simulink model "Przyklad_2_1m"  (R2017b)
settings: Solver=ode45  StartTime=0.0  StopTime=0.05  FixedStep=0.0001  MaxStep=0.0001  RelTol=1e-5  AbsTol=1e-6  EnableMultiTasking=on
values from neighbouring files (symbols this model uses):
  A = [-R2/L 0;0 -1/(R1*(C1+C2))]    [Przyklad_2_1.m]    (also in Przyklad_zs_1.m = [-(1/(R1*C1)+1/(R2*C1)) 1/(R2*C1))
  B = [-A(1,1) 0; 1/(C1+C2) -C2*A(2,2)/(C1+C2)]    [Przyklad_2_1.m]
  C = [1 0;0 -C1*A(2,2);0 C2*A(2,2)]    [Przyklad_2_1.m]
  D = [0 0;-C1*B(2,1) -C1*B(2,2); C2*B(2,1) C2*B(2,2)]    [Przyklad_2_1.m]
  D1 = [0 0;0 -C2*D(2,1);0 C1*D(3,1)]    [Przyklad_2_1.m]

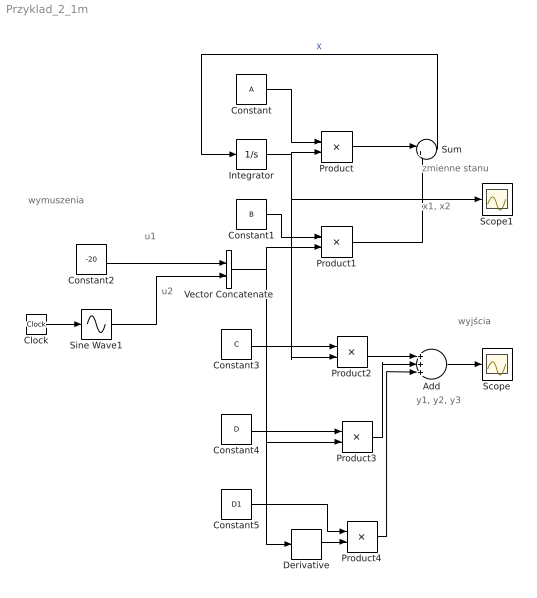
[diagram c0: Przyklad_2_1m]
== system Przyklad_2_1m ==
  note: x1, x2
  note: y1, y2, y3
  note: u2
  note: u1
  note: wymuszenia
  note: wyjścia
  note: zmienne stanu
  Add : Sum  Inputs=+++  SampleTime=0
  Clock : Clock
  Constant : Constant  Value=A  VectorParams1D=off
  Constant1 : Constant  Value=B  VectorParams1D=off
  Constant2 : Constant  Value=-20
  Constant3 : Constant  Value=C  VectorParams1D=off
  Constant4 : Constant  Value=D  VectorParams1D=off
  Constant5 : Constant  Value=D1  VectorParams1D=off
  Derivative : Derivative
  Integrator : Integrator
  Product{,1..4} (5 alike) : Product  Multiplication=Matrix(*)
  Scope : Scope
  Scope1 : Scope
  Sine Wave1 : Sin  TimeSource=Use external signal  Amplitude=50  Frequency=100*pi  SampleTime=0
  Sum : Sum  Inputs=|++
  Vector Concatenate : Concatenate  ConcatenateDimension=2
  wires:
  Integrator/1 -> Product/2, Product2/2, Scope1/1
  Constant/1 -> Product/1
  Constant1/1 -> Product1/1
  Clock/1 -> Sine Wave1/1
  Vector Concatenate/1 -> Product1/2, Derivative/1, Product3/2
  Constant3/1 -> Product2/1
  Derivative/1 -> Product4/2
  Constant5/1 -> Product4/1
  Product/1 -> Sum/1
  Sum/1 -> Integrator/1  "X"
  Product1/1 -> Sum/2
  Constant4/1 -> Product3/1
  Add/1 -> Scope/1
  Product2/1 -> Add/1
  Product3/1 -> Add/2
  Product4/1 -> Add/3
  Sine Wave1/1 -> Vector Concatenate/2
  Constant2/1 -> Vector Concatenate/1
